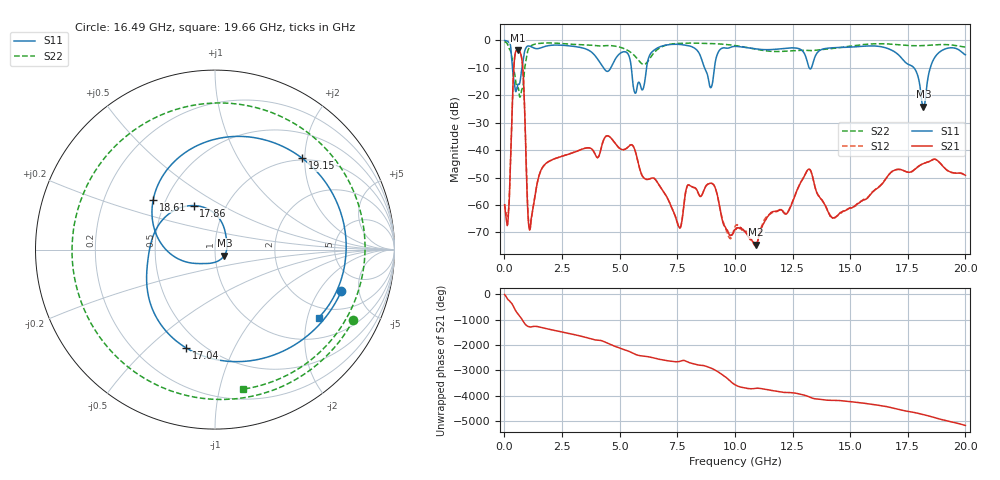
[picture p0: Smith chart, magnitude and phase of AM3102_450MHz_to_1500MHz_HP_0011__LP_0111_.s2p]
!Agilent Technologies,E8364B,MY43040894,A.07.50.67
!Agilent E8364B: A.07.50.67
!Date: Thursday, January 11, 2018 05:31:53
!Correction: S11(Full 2 Port(1,2))
!S21(Full 2 Port(1,2))
!S12(Full 2 Port(1,2))
!S22(Full 2 Port(1,2))
!S2P File: Measurements: S11, S21, S12, S22:
# Hz S  dB  R 50
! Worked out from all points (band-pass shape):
!   1601 points, 10 MHz to 20 GHz, reference 50 ohm
!   highest |S21| = -3.52 dB at 572.2 MHz (marker M1); lowest = -74.5 dB at 10.92 GHz (marker M2)
!   |S21| within 3 dB of the highest: 442.6 MHz to 751.1 MHz (308.5 MHz wide, 51.7 % of centre)
!   lowest |S11| = -24.2 dB at 18.18 GHz (marker M3), VSWR 1.13, Z = 55.4 - j3.66 ohm
!   |S11| at or under -10 dB: 5.508 GHz to 6.168 GHz (659.9 MHz wide, 11.3 % of centre); 8.683 GHz to 9.111 GHz (427.9 MHz wide, 4.81 % of centre); 17.77 GHz to 18.48 GHz (708.9 MHz wide, 3.91 % of centre)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
!   |S22| runs from -20.7 to -0.4 dB; largest |S21 - S12| = 0.0016
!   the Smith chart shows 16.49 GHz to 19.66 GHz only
!   S11 on the Smith chart (normalised r, x): 16.49 GHz: 3.22, -3.28; 17.04 GHz: 0.41, -0.67; 17.86 GHz: 0.71, +0.37; 18.61 GHz: 0.43, +0.30; 19.15 GHz: 0.96, +1.94; 19.66 GHz: 1.62, -2.35
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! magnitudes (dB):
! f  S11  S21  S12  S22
! 10 MHz  0.0  -59.9  -59.6  -0.4
! 172.4 MHz  -0.6  -63.8  -62.4  -2.2
! 572.2 MHz  -16.4  -3.5  -3.5  -17.2
! 784.6 MHz  -8.9  -8.7  -8.7  -17.5
! 1.109 GHz  -2.2  -69.0  -68.3  -2.4
! 3.346 GHz  -2.7  -39.7  -39.8  -1.6
! 5.682 GHz  -19.3  -40.5  -40.5  -5.9
! 6.682 GHz  -2.6  -52.3  -52.3  -3.1
! 8.956 GHz  -17.2  -52.0  -52.1  -1.2
! 10.01 GHz  -2.2  -68.9  -67.8  -1.9
! 10.92 GHz  -3.1  -74.5  -74.6  -3.2
! 13.34 GHz  -9.6  -48.8  -48.8  -3.7
! 14.27 GHz  -2.7  -64.7  -64.5  -3.0
! 16.49 GHz  -2.6  -51.2  -51.1  -1.3
! 16.68 GHz  -3.1  -49.0  -48.9  -1.3
! 17.04 GHz  -4.9  -47.0  -47.1  -1.6
! 17.86 GHz  -11.3  -46.6  -46.6  -2.0
! 18.18 GHz  -24.2  -44.9  -44.9  -1.9
! 18.61 GHz  -7.1  -43.4  -43.4  -1.7
! 19.15 GHz  -3.1  -46.9  -46.9  -1.6
! 19.66 GHz  -3.2  -48.4  -48.4  -2.0
! 20 GHz  -5.3  -49.2  -49.3  -2.4
